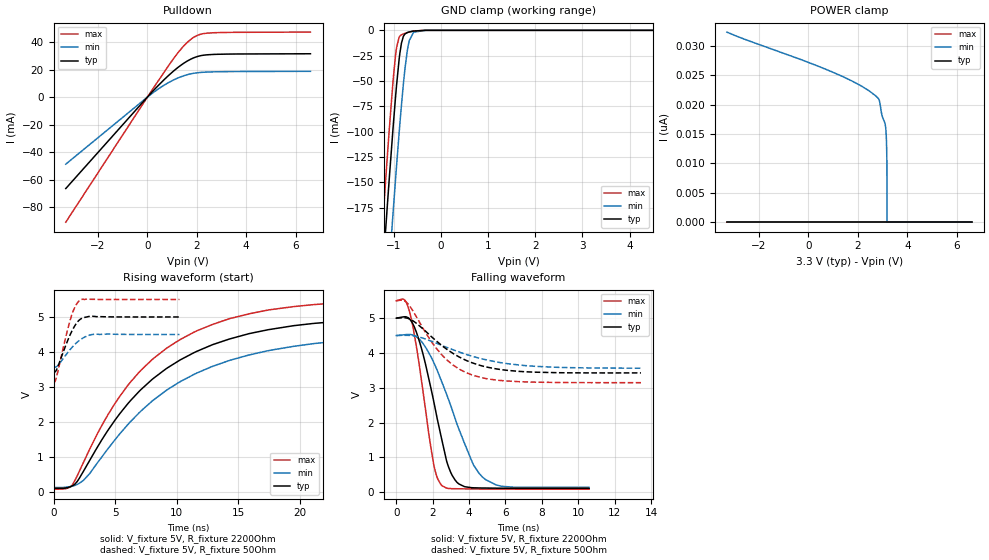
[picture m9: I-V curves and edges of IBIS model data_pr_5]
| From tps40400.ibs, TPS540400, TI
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|   data_pr_5 Model
[Model]   data_pr_5
Model_type   I/O_open_drain
Polarity   Inverting
Vinl = 0.8
Vinh = 2.1
Vmeas = 1.65
Vref = 3.3
Cref = 2pF
Rref = 2200
|   typ   min   max
|   (nom PVT)   (fast PVT)   (slow PVT)
C_comp   1.617e-12   1.585e-12   1.729e-12
| Where nom  PVT is Nominal Process, 3.3V, 25C
|   Fast PVT is Strong Process,  3.4V, -40C
|   Slow PVT is Weak Process,   3.2V, 125C
[Voltage Range]   3.3   3.2   3.4
|Junction Temperature
[Temperature Range]   25   125   -40
[Pullup Reference]   3.3   3.2   3.4
[Pulldown Reference]   0   0   0
[Power Clamp Reference]   3.3   3.2   3.4
[GND Clamp Reference]   0   0   0
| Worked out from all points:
|   slope of the pulldown table from 0 to 0.495 V, typ, clamps not added: 52.4 ohm
|   GND clamp passes 1 mA (typ) near -0.60 V on its own axis
|   falling waveform, V_fixture 5V, R_fixture 2200Ohm: 20-80 % time 1.24ns typ, 1.92ns min, 909ps max; typ from 5 V to 0.112 V
|   rising waveform, V_fixture 5V, R_fixture 2200Ohm: 20-80 % time 8.42ns typ, 9.25ns min, 7.76ns max; typ from 0.112 V to 5 V
|   falling waveform, V_fixture 5V, R_fixture 50Ohm: 20-80 % time 2.57ns typ, 3.39ns min, 2.11ns max; typ from 5 V to 3.43 V
|   rising waveform, V_fixture 5V, R_fixture 50Ohm: 20-80 % time 1.11ns typ, 1.38ns min, 992ps max; typ from 3.43 V to 5 V
[Pulldown]
|   Voltage   I(typ)   I(min)   I(max)
-3.3V     -66.53mA   -48.77mA   -91.01mA
257.4mV   5.028mA    3.596mA    6.933mA
814mV     15.05mA    10.18mA    21.76mA
1.253V    21.83mA    14.09mA    32.62mA
1.48V     24.77mA    15.62mA    37.4mA
1.756V    27.65mA    16.98mA    42.03mA
2.046V    29.71mA    17.82mA    45.17mA
2.439V    30.88mA    18.3mA     46.63mA
6.6V      31.61mA    18.84mA    47.39mA
[GND Clamp]
|   Voltage   I(typ)   I(min)   I(max)
-3.3V     -1.648A    -1.717A    -1.608A
-1.27V    -266.7mA   -355.3mA   -219.2mA
-1.165V   -195.4mA   -282.8mA   -146.8mA
-1.089V   -145.8mA   -231.9mA   -97.3mA
-1.009V   -95.8mA    -179.6mA   -49.55mA
-937mV    -54.97mA   -134.6mA   -17.46mA
-865.6mV  -22.65mA   -92.4mA    -5.675mA
-792mV    -6.034mA   -53.46mA   -3.563mA
-665mV    -1.602mA   -9.956mA   -1.625mA
-573.6mV  -736.5uA   -1.829mA   -633uA
-330.4mV  -7.166uA   -42.24uA   -2.454uA
6.6V      0A         0A         0A
[POWER Clamp]
|   Voltage   I(typ)   I(min)   I(max)
-3.3V     0A         32.36nA    0A
1.253V    0A         25.04nA    0A
2.153V    0A         23.15nA    0A
2.835V    0A         21.01nA    0A
2.886V    0A         20.41nA    0A
2.976V    0A         18.19nA    0A
3.103V    0A         16.67nA    0A
3.138V    0A         15.44nA    0A
3.158V    0A         13.55nA    0A
3.175V    0A         10.01nA    0A
3.177V    0A         0A         0A
6.597V    0A         0A         0A
[Ramp]
R_load = 2200
|   typ   min   max
dV/dt_r   2.93261/8.4301e-09   2.61644/9.26493e-09   3.24557/7.74996e-09
dV/dt_f   2.93273/1.24119e-09   2.61662/1.91561e-09   3.24566/9.08952e-10
[Falling Waveform]
V_fixture = 5V
V_fixture_min = 4.5V
V_fixture_max = 5.5V
R_fixture = 2200Ohm
|   Time   V(typ)   V(min)   V(max)
0s        5V         4.5V       5.5V
480ps     5.04V      4.525V     5.509V
750ps     4.964V     4.53V      5.139V
1.375ns   4.147V     4.332V     3.239V
2.07ns    2.579V     3.713V     759.1mV
2.515ns   1.48V      3.151V     187.1mV
3.34ns    284mV      1.951V     102.3mV
4.245ns   130.2mV    783.7mV    96.66mV
4.9ns     123.2mV    367.5mV    93.52mV
10.6ns    112.2mV    141.7mV    90.62mV
[Rising Waveform]
V_fixture = 5V
V_fixture_min = 4.5V
V_fixture_max = 5.5V
R_fixture = 2200Ohm
|   Time   V(typ)   V(min)   V(max)
0s        112.1mV    138.9mV    90.54mV
1.485ns   178.2mV    173.5mV    194.1mV
2.435ns   602mV      343.1mV    854.1mV
4.43ns    1.772V     1.245V     2.216V
7.135ns   2.939V     2.327V     3.49V
10.26ns   3.769V     3.149V     4.35V
14.26ns   4.367V     3.755V     4.947V
19.54ns   4.753V     4.164V     5.296V
25.43ns   4.919V     4.37V      5.439V
45.36ns   4.997V     4.494V     5.498V
[Falling Waveform]
V_fixture = 5V
V_fixture_min = 4.5V
V_fixture_max = 5.5V
R_fixture = 50Ohm
|   Time   V(typ)   V(min)   V(max)
0s        5V         4.5V       5.5V
390ps     5.011V     4.507V     5.51V
625ps     4.996V     4.506V     5.42V
1.975ns   4.446V     4.328V     4.292V
2.78ns    4.105V     4.159V     3.801V
3.43ns    3.893V     4.033V     3.547V
4.27ns    3.7V       3.891V     3.352V
5.495ns   3.543V     3.744V     3.222V
7.09ns    3.461V     3.637V     3.17V
13.45ns   3.428V     3.562V     3.147V
[Rising Waveform]
V_fixture = 5V
V_fixture_min = 4.5V
V_fixture_max = 5.5V
R_fixture = 50Ohm
|   Time   V(typ)   V(min)   V(max)
0s        3.43V      3.567V     3.144V
115ps     3.433V     3.567V     3.16V
235ps     3.488V     3.581V     3.279V
1.085ns   4.271V     3.954V     4.558V
1.495ns   4.598V     4.129V     5.072V
1.86ns    4.819V     4.262V     5.359V
2.21ns    4.944V     4.359V     5.491V
2.85ns    5.013V     4.474V     5.51V
3.44ns    5.012V     4.51V      5.502V
10.24ns   5V         4.5V       5.5V
